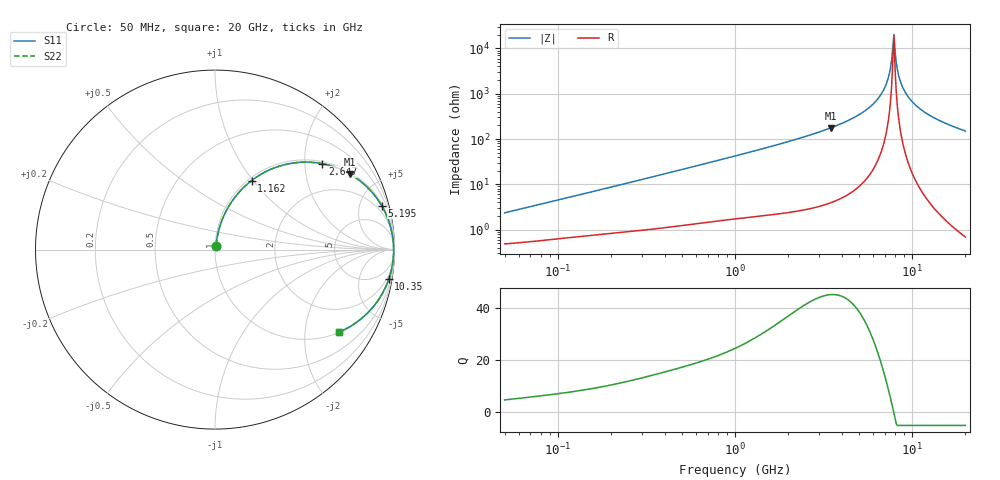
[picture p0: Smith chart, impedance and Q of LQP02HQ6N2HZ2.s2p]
!Murata Part Number: LQP02HQ6N2HZ2
!These Parameters are Measured in Series Mode Connection
!  o--[Z]--o
!Port1  Port2
!  o-------o
!Freq. Start=50[MHz] Stop=20[GHz], 401[Steps]
# Hz S RI R 50
!Freq.(Hz) S11(Real) S11(Imag) S21(Real) S21(Imag) S12(Real) S12(Imag) S22(Real) S22(Imag)
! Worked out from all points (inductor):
!   401 points, 50 MHz to 20 GHz, reference 50 ohm
!   read as one part in series: L = 7.27 nH near 51.52 MHz
!   highest Q = 45 at 3.467 GHz (marker M1), where L = 8.1 nH
!   self-resonance near 7.784 GHz
!   S11 on the Smith chart (normalised r, x): 50 MHz: 1.01, +0.05; 1.162 GHz: 1.04, +0.98; 2.647 GHz: 1.06, +2.45; 5.195 GHz: 1.20, +7.53; 10.35 GHz: 1, -12; 20 GHz: 1.01, -3.01
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5e7  0.00535 0.0228  0.9946 -0.0228  0.9946 -0.0228  0.00535 0.0228
1.364002e8  0.0106 0.0592  0.9894 -0.0592  0.9894 -0.0592  0.0106 0.0592
3.721004e8  0.0344 0.1518  0.9656 -0.1518  0.9656 -0.1518  0.0344 0.1518
1e9  0.1618 0.3483  0.8382 -0.3483  0.8382 -0.3483  0.1618 0.3483
1.161586e9  0.2042 0.3848  0.7958 -0.3848  0.7958 -0.3848  0.2042 0.3848
2.647493e9  0.5985 0.4785  0.4015 -0.4785  0.4015 -0.4785  0.5985 0.4785
2.728004e9  0.6161 0.4748  0.3839 -0.4748  0.3839 -0.4748  0.6161 0.4748
3.466789e9  0.7521 0.4208  0.2479 -0.4208  0.2479 -0.4208  0.7521 0.4208
5.194772e9  0.9284 0.2447  0.0716 -0.2447  0.0716 -0.2447  0.9284 0.2447
6.601595e9  0.9827 0.1078  0.0173 -0.1078  0.0173 -0.1078  0.9827 0.1078
7.114996e9  0.9909 0.0626  0.00905 -0.0626  0.00905 -0.0626  0.9909 0.0626
7.442007e9  0.9939 0.0352  0.00614 -0.0352  0.00614 -0.0352  0.9939 0.0352
7.668323e9  0.9949 0.0169  0.00506 -0.0169  0.00506 -0.0169  0.9949 0.0169
7.901521e9  0.9953 -0.00149  0.00465 0.00149  0.00465 0.00149  0.9953 -0.00149
8.020766e9  0.9953 -0.0107  0.00471 0.0107  0.00471 0.0107  0.9953 -0.0107
8.141811e9  0.9951 -0.0199  0.00494 0.0199  0.00494 0.0199  0.9951 -0.0199
8.389408e9  0.9941 -0.0382  0.0059 0.0382  0.0059 0.0382  0.9941 -0.0382
8.774992e9  0.9914 -0.0657  0.00864 0.0657  0.00864 0.0657  0.9914 -0.0657
9.457416e9  0.9834 -0.111  0.0166 0.111  0.0166 0.111  0.9834 -0.111
1.034674e10  0.9682 -0.1644  0.0318 0.1644  0.0318 0.1644  0.9682 -0.1644
1.354865e10  0.8874 -0.3113  0.1126 0.3113  0.1126 0.3113  0.8874 -0.3113
2e10  0.6936 -0.4587  0.3064 0.4587  0.3064 0.4587  0.6936 -0.4587
